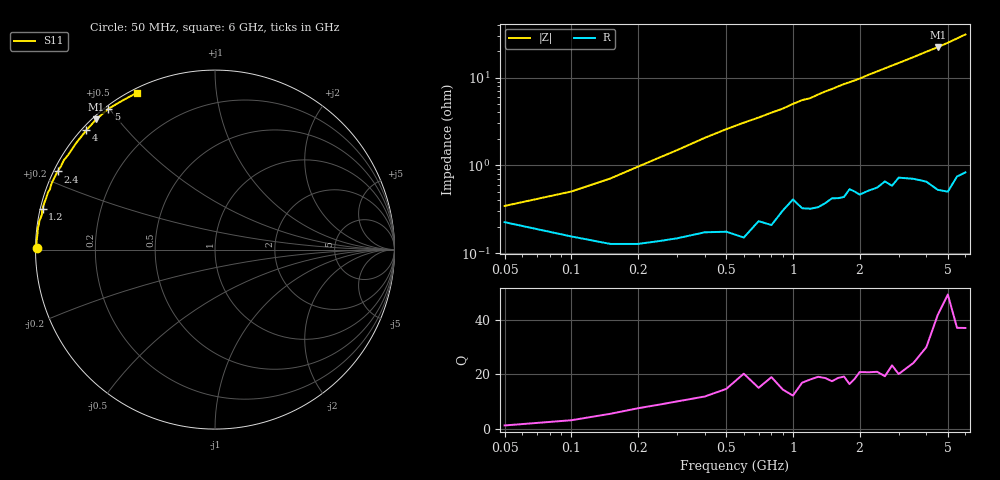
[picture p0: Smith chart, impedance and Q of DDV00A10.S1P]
! Infineon Technologies  Discrete & RF Semiconductors
! BBY58-02W
! Si Tuning Diode in SCD-80
! VR =
! S-Parameters:  June  2000
# GHz  S  MA  R  50
!  f  S11
! GHz  MAG  ANG
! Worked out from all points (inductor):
!   34 points, 50 MHz to 6 GHz, reference 50 ohm
!   read as one part to ground: L = 764 pH near 100 MHz
!   highest Q = 41.9 at 4.5 GHz (marker M1), where L = 782 pH
!   S11 on the Smith chart (normalised r, x): 50 MHz: 0.00, +0.01; 1.2 GHz: 0.01, +0.12; 2.4 GHz: 0.01, +0.23; 4 GHz: 0.01, +0.39; 5 GHz: 0.01, +0.50; 6 GHz: 0.02, +0.62
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0.05  0.991 179.4
0.1  0.9938 178.9
0.2  0.9949 177.8
0.5  0.993 174.1
0.6  0.994 173.0
0.7  0.9908 172.0
0.8  0.9917 170.9
0.9  0.9879 169.9
1  0.9839 168.6
1.1  0.9872 167.4
1.2  0.9874 166.7
1.4  0.9855 164.2
1.5  0.9836 163.2
1.6  0.9836 162.0
1.7  0.9831 160.9
1.8  0.9794 160.0
2  0.9822 158.0
2.2  0.9804 155.7
2.4  0.979 153.6
2.6  0.9756 151.5
2.8  0.9784 149.4
3  0.9736 147.4
3.5  0.9751 142.3
4  0.9776 137.1
4.5  0.9825 132.3
5  0.984 127.1
5.5  0.9774 121.8
6  0.9762 116.6
